| TEXAS INSTRUMENTS INCORPORATED
| Standard Linear and Logic Group
| IBIS Model of sn74lvch162244a
| 16 BIT BUFFER/DRIVER WITH 3-STATE OUTPUTS
| This file contains package information for the following:
|  SSOP 48-pin (DL) package as [Component] lvch162244a_DL
|  TSSOP 48-pin (DGG) package as [Component] lvch162244a_DGG
|  TVSOP 48-pin (DGV) package as [Component] lvch162244a_DGV
| This device can be powered at the following Vccs:
|  1.8 volt Vcc
|  2.5 volt Vcc
|  3.3 volt Vcc
| This file provides unique models under the [Model Selector] for each Vcc.
| For operation at a specific Vcc, select the appropriate model after each
| [Model Selector] keyword.
[IBIS Ver]   3.2
[Comment char]  |_char
[File Name]   sn74lvch162244a.ibs
[File Rev]   1.1 | e_die
[Date]   March 9, 2002
[Source]   Data created from TI-SPICE simulations at TI-SLL.
[Notes]   The following is an IBIS list for the lvch162244a.
   Please contact sllibis@ti.com with questions and
   comments concerning SLL IBIS models.
   This IBIS model is created from a BA (back annotated netlist
   Non-monotonic data input model due to bushold
   Non-monotonic data output model due to damping resistor.
   C_comp values are taken at a different test condition than
   the data sheet.
[Disclaimer] Property of Texas Instruments Incorporated.  Unauthorized
   reproduction and/or distribution is strictly prohibited.
   This product is protected under copyright law.
   Created  2002, (C) Copyright  2002, Texas Instruments
   Incorporated, All Rights Reserved
   UNLESS THERE IS A SIGNED, WRITTEN AGREEMENT TO THE
   CONTRARY, TEXAS INSTRUMENTS (TI) IS PROVIDING THE IBIS
   MODELS  AND WITHOUT ANY WARRANTY, EXPRESSED OR
   IMPLIED.  TI assumes no liability for:
   1) the accuracy of the IBIS models provided to your
   company;
   2) the proper functioning of these IBIS Models in your
   design or for any resulting applications; or
   3) infringement of patents, copyrights or intellectual
   property rights resulting from your use of these IBIS
   models.
   TI provides IBIS Models as a service to our customers.
   You and your company shall not distribute, sell or give
   these models to anyone else without prior written
   permission from TI.
   TI reserves the right to make changes to our products or
   to discontinue any semiconductor product or service
   without notice, and advises our customers to obtain the
   latest version of relevant information to verify, before
   placing orders, that the information being relied on is
   current.
   Please be aware that your receipt and use of the IBIS
   information provided shall serve as acceptance of these
   terms and conditions.  If you do not accept these terms,
   you should return or destroy the IBIS models and any
   other accompanying information immediately.
| Component lvch162244a_DL 48-pin SSOP
[Component]   lvch162244a_DL
[Manufacturer]   Texas Instruments, Inc.
[Package]
|   typ   min   max
R_pkg   4.800e-02   3.800e-02   5.300e-02
L_pkg   6.046e-09   5.084e-09   7.968e-09
C_pkg   8.130e-13   5.690e-13   1.157e-12
[Pin]   signal_name   model_name   R_pin   L_pin   C_pin
1   1OE_BAR   lvch162244a_NOE   4.600e-02   7.968e-09   1.017e-12
2   1Y1   lvch162244a_OUT   4.400e-02   7.299e-09   1.157e-12
3   1Y2   lvch162244a_OUT   4.300e-02   6.765e-09   1.058e-12
4   GND   GND   4.100e-02   6.269e-09   9.330e-13
5   1Y3   lvch162244a_OUT   3.800e-02   5.856e-09   8.290e-13
6   1Y4   lvch162244a_OUT   4.600e-02   5.802e-09   7.900e-13
7   VCC   POWER   5.000e-02   5.656e-09   7.380e-13
8   2Y1   lvch162244a_OUT   5.300e-02   5.500e-09   6.430e-13
9   2Y2   lvch162244a_OUT   5.200e-02   5.304e-09   6.060e-13
10   GND   GND   5.300e-02   5.189e-09   5.830e-13
11   2Y3   lvch162244a_OUT   5.100e-02   5.084e-09   5.690e-13
12   2Y4   lvch162244a_OUT   5.300e-02   5.862e-09   8.330e-13
13   3Y1   lvch162244a_OUT   5.300e-02   5.862e-09   8.330e-13
14   3Y2   lvch162244a_OUT   5.100e-02   5.084e-09   5.690e-13
15   GND   GND   5.300e-02   5.189e-09   5.830e-13
16   3Y3   lvch162244a_OUT   5.200e-02   5.304e-09   6.060e-13
17   3Y4   lvch162244a_OUT   5.300e-02   5.500e-09   6.430e-13
18   VCC   POWER   5.000e-02   5.656e-09   7.380e-13
19   4Y1   lvch162244a_OUT   4.600e-02   5.802e-09   7.900e-13
20   4Y2   lvch162244a_OUT   3.800e-02   5.856e-09   8.290e-13
21   GND   GND   4.100e-02   6.269e-09   9.330e-13
22   4Y3   lvch162244a_OUT   4.300e-02   6.765e-09   1.058e-12
23   4Y4   lvch162244a_OUT   4.400e-02   7.299e-09   1.157e-12
24   40E_BAR   lvch162244a_NOE   4.600e-02   7.968e-09   1.017e-12
25   3OE_BAR   lvch162244a_NOE   4.600e-02   7.968e-09   1.017e-12
26   4A4   lvch162244a_IN   4.400e-02   7.299e-09   1.157e-12
27   4A3   lvch162244a_IN   4.300e-02   6.765e-09   1.058e-12
28   GND   GND   4.100e-02   6.269e-09   9.330e-13
29   4A2   lvch162244a_IN   3.800e-02   5.856e-09   8.290e-13
30   4A1   lvch162244a_IN   4.600e-02   5.802e-09   7.900e-13
31   VCC   POWER   5.000e-02   5.656e-09   7.380e-13
32   3A4   lvch162244a_IN   5.300e-02   5.500e-09   6.430e-13
33   3A3   lvch162244a_IN   5.200e-02   5.304e-09   6.060e-13
34   GND   GND   5.300e-02   5.189e-09   5.830e-13
35   3A2   lvch162244a_IN   5.100e-02   5.084e-09   5.690e-13
36   3A1   lvch162244a_IN   5.300e-02   5.862e-09   8.330e-13
37   2A4   lvch162244a_IN   5.300e-02   5.862e-09   8.330e-13
38   2A3   lvch162244a_IN   5.100e-02   5.084e-09   5.690e-13
39   GND   GND   5.300e-02   5.189e-09   5.830e-13
40   2A2   lvch162244a_IN   5.200e-02   5.304e-09   6.060e-13
41   2A1   lvch162244a_IN   5.300e-02   5.500e-09   6.430e-13
42   VCC   POWER   5.000e-02   5.656e-09   7.380e-13
43   1A4   lvch162244a_IN   4.600e-02   5.802e-09   7.900e-13
44   1A3   lvch162244a_IN   3.800e-02   5.856e-09   8.290e-13
45   GND   GND   4.100e-02   6.269e-09   9.330e-13
46   1A2   lvch162244a_IN   4.300e-02   6.765e-09   1.058e-12
47   1A1   lvch162244a_IN   4.400e-02   7.299e-09   1.157e-12
48   2OE_BAR   lvch162244a_NOE   4.600e-02   7.967e-09   1.017e-12
| Component lvch162244a_DGG 48-pin TSSOP
[Component]   lvch162244a_DGG
[Manufacturer]   Texas Instruments, Inc.
[Package]
|   typ   min   max
R_pkg   4.400e-02   3.800e-02   5.100e-02
L_pkg   3.019e-09   2.486e-09   4.099e-09
C_pkg   5.070e-13   3.340e-13   8.090e-13
[Pin]   signal_name   model_name   R_pin   L_pin   C_pin
1   1OE_BAR   lvch162244a_NOE   4.100e-02   4.017e-09   7.590e-13
2   1Y1   lvch162244a_OUT   4.200e-02   3.737e-09   7.920e-13
3   1Y2   lvch162244a_OUT   4.200e-02   3.480e-09   6.610e-13
4   GND   GND   3.800e-02   3.131e-09   5.750e-13
5   1Y3   lvch162244a_OUT   4.700e-02   3.122e-09   5.660e-13
6   1Y4   lvch162244a_OUT   4.300e-02   2.948e-09   5.040e-13
7   VCC   POWER   4.500e-02   2.845e-09   3.970e-13
8   2Y1   lvch162244a_OUT   4.900e-02   2.835e-09   3.940e-13
9   2Y2   lvch162244a_OUT   4.800e-02   2.715e-09   3.780e-13
10   GND   GND   5.000e-02   2.664e-09   3.630e-13
11   2Y3   lvch162244a_OUT   5.000e-02   2.585e-09   3.480e-13
12   2Y4   lvch162244a_OUT   4.900e-02   2.550e-09   3.370e-13
13   3Y1   lvch162244a_OUT   4.900e-02   2.541e-09   3.360e-13
14   3Y2   lvch162244a_OUT   5.000e-02   2.574e-09   3.480e-13
15   GND   GND   4.900e-02   2.618e-09   3.590e-13
16   3Y3   lvch162244a_OUT   4.600e-02   2.671e-09   3.750e-13
17   3Y4   lvch162244a_OUT   4.500e-02   2.754e-09   3.890e-13
18   VCC   POWER   4.400e-02   2.823e-09   4.500e-13
19   4Y1   lvch162244a_OUT   4.200e-02   2.968e-09   5.030e-13
20   4Y2   lvch162244a_OUT   5.100e-02   3.108e-09   5.350e-13
21   GND   GND   4.200e-02   3.175e-09   5.870e-13
22   4Y3   lvch162244a_OUT   4.100e-02   3.449e-09   6.780e-13
23   4Y4   lvch162244a_OUT   4.400e-02   3.766e-09   8.040e-13
24   40E_BAR   lvch162244a_NOE   4.300e-02   4.065e-09   7.610e-13
25   3OE_BAR   lvch162244a_NOE   4.100e-02   3.994e-09   7.570e-13
26   4A4   lvch162244a_IN   3.900e-02   3.649e-09   7.890e-13
27   4A3   lvch162244a_IN   3.800e-02   3.362e-09   6.600e-13
28   GND   GND   3.800e-02   3.082e-09   5.740e-13
29   4A2   lvch162244a_IN   4.400e-02   2.990e-09   5.220e-13
30   4A1   lvch162244a_IN   4.100e-02   2.917e-09   4.950e-13
31   VCC   POWER   4.300e-02   2.820e-09   4.480e-13
32   3A4   lvch162244a_IN   4.300e-02   2.699e-09   3.850e-13
33   3A3   lvch162244a_IN   4.500e-02   2.628e-09   3.720e-13
34   GND   GND   4.600e-02   2.556e-09   3.560e-13
35   3A2   lvch162244a_IN   4.600e-02   2.495e-09   3.440e-13
36   3A1   lvch162244a_IN   4.700e-02   2.487e-09   3.340e-13
37   2A4   lvch162244a_IN   4.700e-02   2.490e-09   3.350e-13
38   2A3   lvch162244a_IN   4.600e-02   2.486e-09   3.430e-13
39   GND   GND   4.500e-02   2.566e-09   3.560e-13
40   2A2   lvch162244a_IN   4.400e-02   2.639e-09   3.740e-13
41   2A1   lvch162244a_IN   4.300e-02   2.701e-09   3.860e-13
42   VCC   POWER   4.300e-02   2.817e-09   4.500e-13
43   1A4   lvch162244a_IN   4.100e-02   2.935e-09   5.010e-13
44   1A3   lvch162244a_IN   4.700e-02   3.035e-09   5.290e-13
45   GND   GND   4.300e-02   3.171e-09   5.890e-13
46   1A2   lvch162244a_IN   4.000e-02   3.415e-09   6.820e-13
47   1A1   lvch162244a_IN   4.300e-02   3.741e-09   8.090e-13
48   2OE_BAR   lvch162244a_NOE   4.400e-02   4.099e-09   7.640e-13
| Component lvch162244a_DGV 48-pin TVSOP
[Component]   lvch162244a_DGV
[Manufacturer]   Texas Instruments, Inc.
[Package]
|   typ   min   max
R_pkg   7.000e-02   4.900e-02   8.500e-02
L_pkg   3.013e-09   2.743e-09   3.408e-09
C_pkg   3.710e-13   2.940e-13   5.110e-13
[Pin]   signal_name   model_name   R_pin   L_pin   C_pin
1   1OE_BAR   lvch162244a_NOE   4.900e-02   3.393e-09   4.970e-13
2   1Y1   lvch162244a_OUT   6.000e-02   3.250e-09   5.020e-13
3   1Y2   lvch162244a_OUT   7.700e-02   3.310e-09   4.510e-13
4   GND   GND   8.500e-02   3.299e-09   4.040e-13
5   1Y3   lvch162244a_OUT   8.300e-02   3.136e-09   3.600e-13
6   1Y4   lvch162244a_OUT   7.700e-02   3.019e-09   3.630e-13
7   VCC   POWER   6.500e-02   2.882e-09   3.490e-13
8   2Y1   lvch162244a_OUT   6.600e-02   2.829e-09   3.140e-13
9   2Y2   lvch162244a_OUT   6.700e-02   2.796e-09   3.140e-13
10   GND   GND   6.900e-02   2.754e-09   3.080e-13
11   2Y3   lvch162244a_OUT   7.000e-02   2.753e-09   3.010e-13
12   2Y4   lvch162244a_OUT   7.100e-02   2.745e-09   2.940e-13
13   3Y1   lvch162244a_OUT   7.000e-02   2.744e-09   2.940e-13
14   3Y2   lvch162244a_OUT   7.000e-02   2.754e-09   3.010e-13
15   GND   GND   6.900e-02   2.754e-09   3.080e-13
16   3Y3   lvch162244a_OUT   6.700e-02   2.796e-09   3.140e-13
17   3Y4   lvch162244a_OUT   6.600e-02   2.829e-09   3.140e-13
18   VCC   POWER   6.500e-02   2.883e-09   3.500e-13
19   4Y1   lvch162244a_OUT   7.500e-02   3.014e-09   3.630e-13
20   4Y2   lvch162244a_OUT   8.000e-02   3.128e-09   3.580e-13
21   GND   GND   8.400e-02   3.295e-09   4.030e-13
22   4Y3   lvch162244a_OUT   7.800e-02   3.311e-09   4.520e-13
23   4Y4   lvch162244a_OUT   6.200e-02   3.259e-09   5.010e-13
24   40E_BAR   lvch162244a_NOE   5.200e-02   3.404e-09   4.960e-13
25   3OE_BAR   lvch162244a_NOE   5.300e-02   3.397e-09   5.050e-13
26   4A4   lvch162244a_IN   6.200e-02   3.249e-09   5.110e-13
27   4A3   lvch162244a_IN   7.700e-02   3.308e-09   4.530e-13
28   GND   GND   8.200e-02   3.289e-09   4.030e-13
29   4A2   lvch162244a_IN   7.800e-02   3.121e-09   3.590e-13
30   4A1   lvch162244a_IN   7.400e-02   3.010e-09   3.630e-13
31   VCC   POWER   6.500e-02   2.883e-09   3.490e-13
32   3A4   lvch162244a_IN   6.700e-02   2.829e-09   3.140e-13
33   3A3   lvch162244a_IN   6.700e-02   2.795e-09   3.140e-13
34   GND   GND   6.900e-02   2.753e-09   3.070e-13
35   3A2   lvch162244a_IN   7.000e-02   2.753e-09   3.010e-13
36   3A1   lvch162244a_IN   7.000e-02   2.743e-09   2.940e-13
37   2A4   lvch162244a_IN   7.000e-02   2.743e-09   2.940e-13
38   2A3   lvch162244a_IN   7.000e-02   2.753e-09   3.010e-13
39   GND   GND   6.900e-02   2.754e-09   3.070e-13
40   2A2   lvch162244a_IN   6.800e-02   2.797e-09   3.140e-13
41   2A1   lvch162244a_IN   6.700e-02   2.830e-09   3.140e-13
42   VCC   POWER   6.400e-02   2.880e-09   3.490e-13
43   1A4   lvch162244a_IN   7.200e-02   3.004e-09   3.620e-13
44   1A3   lvch162244a_IN   7.800e-02   3.121e-09   3.590e-13
45   GND   GND   8.400e-02   3.296e-09   4.030e-13
46   1A2   lvch162244a_IN   7.700e-02   3.308e-09   4.510e-13
47   1A1   lvch162244a_IN   6.200e-02   3.258e-09   4.990e-13
48   2OE_BAR   lvch162244a_NOE   5.300e-02   3.408e-09   4.940e-13
| Model lvch162244a_NOE
[Model Selector]   lvch162244a_NOE
lvch162244a_NOE_18   1.8 volt Vcc
lvch162244a_NOE_25   2.5 volt Vcc
lvch162244a_NOE_33   3.3 volt Vcc
| Model lvch162244a_IN
[Model Selector]   lvch162244a_IN
lvch162244a_IN_18   1.8 volt Vcc
lvch162244a_IN_25   2.5 volt Vcc
lvch162244a_IN_33   3.3 volt Vcc
| Model lvch162244a_OUT
[Model Selector]   lvch162244a_OUT
lvch162244a_OUT_18   1.8 volt Vcc
lvch162244a_OUT_25   2.5 volt Vcc
lvch162244a_OUT_33   3.3 volt Vcc
| Models and submodels in the file (9): lvch162244a_NOE_18 (Input), lvch162244a_NOE_25 (Input), lvch162244a_NOE_33 (Input), lvch162244a_IN_18 (Input), lvch162244a_IN_25 (Input), lvch162244a_IN_33 (Input), lvch162244a_OUT_18 (3-state), lvch162244a_OUT_25 (3-state), lvch162244a_OUT_33 (3-state)
